(* Logix 5000 AddOnInstructionDefinition export Banner_T30R_Q90R_KD_PD_v4; software revision 33.00 *)

TYPE Banner_T30R_Q90R_KD_PDI0_v4 :   // Process Data for a T30R or Q90R sensors. Digital Measurement Data Set.
STRUCT
   Measurement : DINT;   // Distance Measurement Value
   Scale : DINT;   // Scale Factor for Measurement
   Stability : SINT;   // 0 = No target or marginal signal 1 = Valid
   BDC1_State : SINT;   // 0 = Inactive 1 = Active
   BDC2_State : INT;   // 0 = Inactive 1 = Active
END_STRUCT
END_TYPE

TYPE Banner_T30R_Q90R_KD_PDI1_v4 :   // Process Data for a T30R or Q90R sensors. Distance and Excess Gain data set.
STRUCT
   Measurement : DINT;   // Distance Measurement Value
   Excess_Gain : DINT;   // Excess Gain Measurement Value
END_STRUCT
END_TYPE

TYPE Banner_T30R_Q90R_KD_PDI2_v4 :   // Process Data for a T30R or Q90R sensors. Distance and Excess Gain with Binary data set.
STRUCT
   Measurement : DINT;   // Distance Measurement Value
   Excess_Gain : DINT;   // Excess Data Excess Gain Measurement
   Stability : SINT;   // 0 = No traget or marginal signal, 1 = Valid
   BDC1_State : SINT;   // 0 = Inactive 1 = Active
   BDC2_State : INT;   // 0 = Inactive 1 = Active
END_STRUCT
END_TYPE

TYPE Banner_T30R_Q90R_KD_PDI_v4 :   // Process Data for a T30R or Q90R sensors.
STRUCT
   Set_0 : Banner_T30R_Q90R_KD_PDI0_v4;
   Set_1 : Banner_T30R_Q90R_KD_PDI1_v4;
   Set_2 : Banner_T30R_Q90R_KD_PDI2_v4;
   PDI_DT : SINT[6];
END_STRUCT
END_TYPE

ADD_ON_INSTRUCTION Banner_T30R_Q90R_KD_PD_v4   (* revision 4.0, vendor Banner Engineering *)
// Take raw process data and convert it to usable values.
VAR_IN_OUT
   Process_Data : Banner_T30R_Q90R_KD_PDI_v4; {required}
END_VAR
VAR_INPUT
   Process_Data_Layout : SINT; {required}
   Byte_Swap : BOOL; {required}
END_VAR
VAR
   Temp : SINT[6]; {access None}
END_VAR

ROUTINE Logic   (* ladder *)
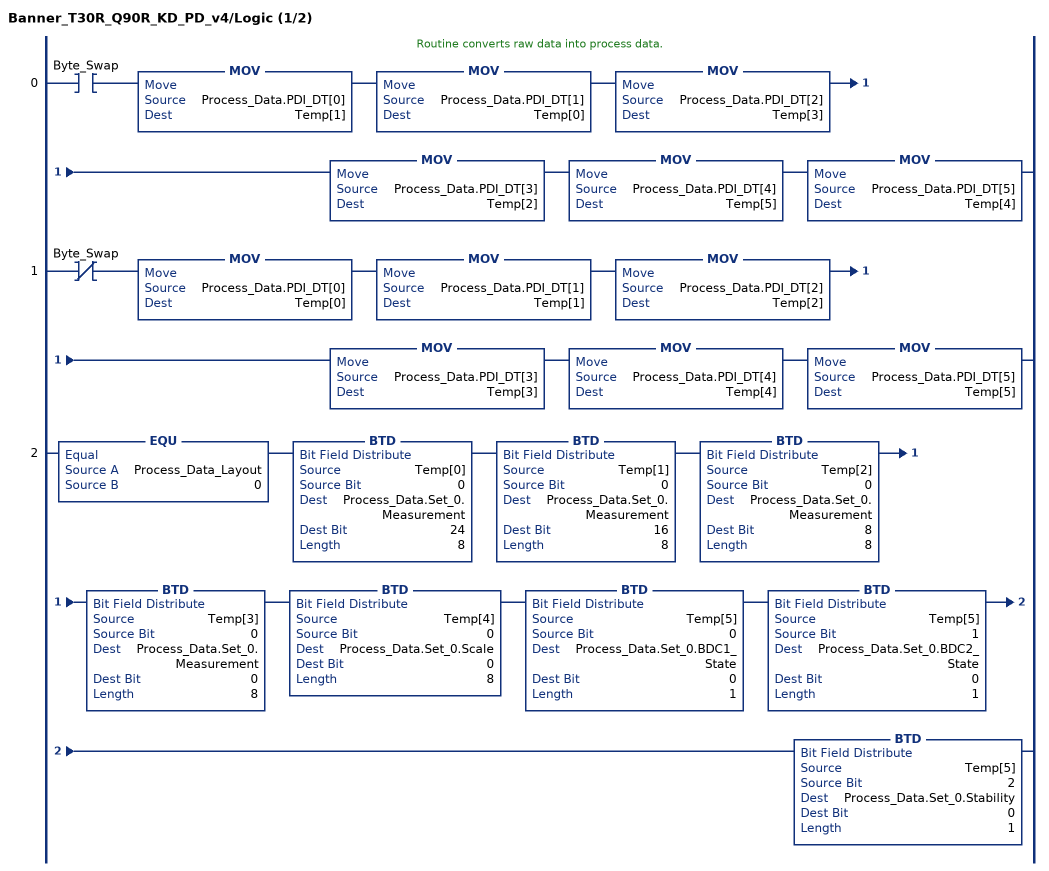
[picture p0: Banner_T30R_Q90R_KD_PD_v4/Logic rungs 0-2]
   // Routine converts raw data into process data.
   0: XIC(Byte_Swap)MOV(Process_Data.PDI_DT[0],Temp[1])MOV(Process_Data.PDI_DT[1],Temp[0])MOV(Process_Data.PDI_DT[2],Temp[3])MOV(Process_Data.PDI_DT[3],Temp[2])MOV(Process_Data.PDI_DT[4],Temp[5])MOV(Process_Data.PDI_DT[5],Temp[4]);
   1: XIO(Byte_Swap)MOV(Process_Data.PDI_DT[0],Temp[0])MOV(Process_Data.PDI_DT[1],Temp[1])MOV(Process_Data.PDI_DT[2],Temp[2])MOV(Process_Data.PDI_DT[3],Temp[3])MOV(Process_Data.PDI_DT[4],Temp[4])MOV(Process_Data.PDI_DT[5],Temp[5]);
   2: EQU(Process_Data_Layout,0)BTD(Temp[0],0,Process_Data.Set_0.Measurement,24,8)BTD(Temp[1],0,Process_Data.Set_0.Measurement,16,8)BTD(Temp[2],0,Process_Data.Set_0.Measurement,8,8)BTD(Temp[3],0,Process_Data.Set_0.Measurement,0,8)BTD(Temp[4],0,Process_Data.Set_0.Scale,0,8)BTD(Temp[5],0,Process_Data.Set_0.BDC1_State,0,1)BTD(Temp[5],1,Process_Data.Set_0.BDC2_State,0,1)BTD(Temp[5],2,Process_Data.Set_0.Stability,0,1);
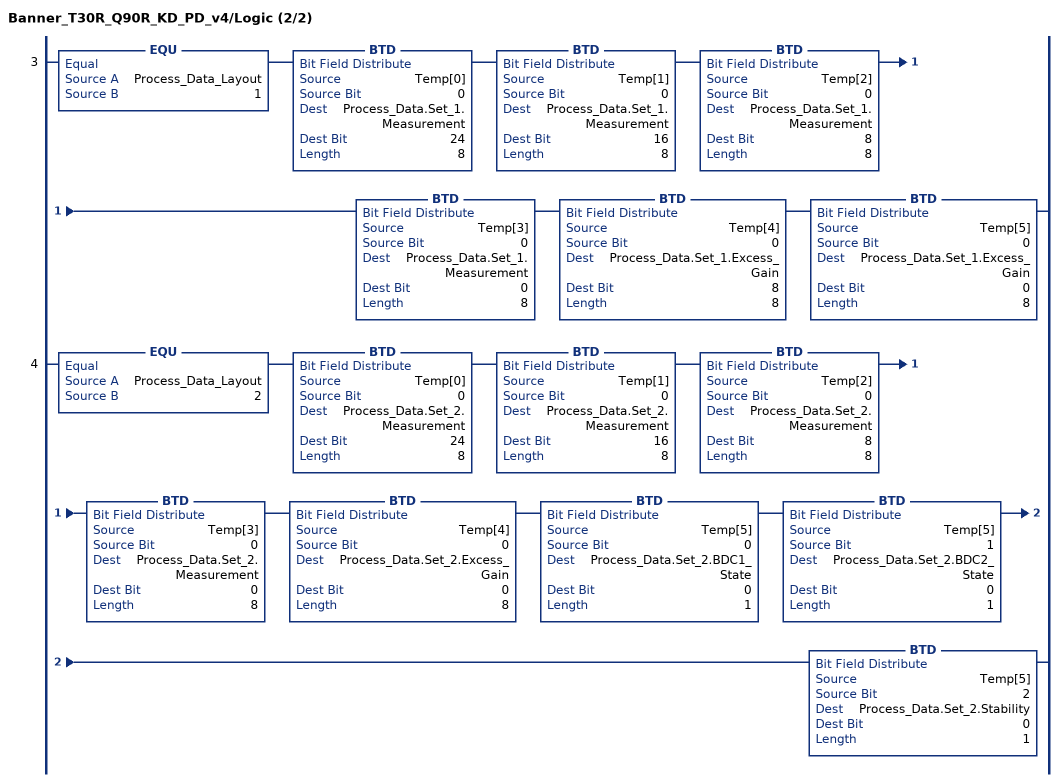
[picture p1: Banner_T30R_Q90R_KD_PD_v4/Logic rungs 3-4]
   3: EQU(Process_Data_Layout,1)BTD(Temp[0],0,Process_Data.Set_1.Measurement,24,8)BTD(Temp[1],0,Process_Data.Set_1.Measurement,16,8)BTD(Temp[2],0,Process_Data.Set_1.Measurement,8,8)BTD(Temp[3],0,Process_Data.Set_1.Measurement,0,8)BTD(Temp[4],0,Process_Data.Set_1.Excess_Gain,8,8)BTD(Temp[5],0,Process_Data.Set_1.Excess_Gain,0,8);
   4: EQU(Process_Data_Layout,2)BTD(Temp[0],0,Process_Data.Set_2.Measurement,24,8)BTD(Temp[1],0,Process_Data.Set_2.Measurement,16,8)BTD(Temp[2],0,Process_Data.Set_2.Measurement,8,8)BTD(Temp[3],0,Process_Data.Set_2.Measurement,0,8)BTD(Temp[4],0,Process_Data.Set_2.Excess_Gain,0,8)BTD(Temp[5],0,Process_Data.Set_2.BDC1_State,0,1)BTD(Temp[5],1,Process_Data.Set_2.BDC2_State,0,1)BTD(Temp[5],2,Process_Data.Set_2.Stability,0,1);
END_ROUTINE
END_ADD_ON_INSTRUCTION
